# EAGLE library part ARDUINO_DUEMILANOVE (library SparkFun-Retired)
Arduino Duemilanove Shield Footprint Shield form compatible with the Arduino Duemilanove.
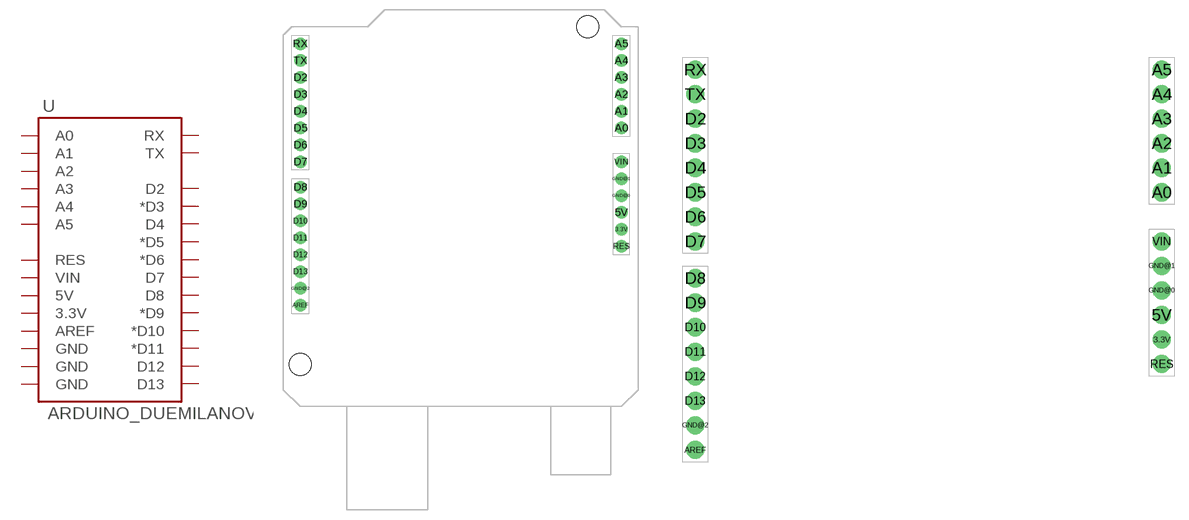
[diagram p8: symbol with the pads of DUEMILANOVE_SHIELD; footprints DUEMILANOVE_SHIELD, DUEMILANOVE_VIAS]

Designator prefix U

## ARDUINO_DUEMILANOVELABEL  [DUEMILANOVE_SHIELD]
3.3V  3.3V
5V  5V
A0  A0
A1  A1
A2  A2
A3  A3
A4  A4
A5  A5
AREF  AREF
D2  D2
D3  *D3
D4  D4
D5  *D5
D6  *D6
D7  D7
D8  D8
D9  *D9
D10  *D10
D11  *D11
D12  D12
D13  D13
GND@0  GND
GND@1  GND
GND@2  GND
RES  RES
RX  RX
TX  TX
VIN  VIN

## ARDUINO_DUEMILANOVENO_SILK  [DUEMILANOVE_VIAS]
Pads as for DUEMILANOVE_SHIELD

## ARDUINO_DUEMILANOVENOHOLES  [DUEMILANOVE_SHIELD_NOHOLES]
Pads as for DUEMILANOVE_SHIELD

## ARDUINO_DUEMILANOVELONGPADS  [DUEMILANOVE_SHIELD_LONGPADS]
Pads as for DUEMILANOVE_SHIELD

## ARDUINO_DUEMILANOVENOLABELS  [DUEMILANOVE_SHIELD_NOLABELS]
Pads as for DUEMILANOVE_SHIELD

## ARDUINO_DUEMILANOVENOHOLESORLABELS  [DUEMILANOVE_SHIELD_NOHOLES_NOLABELS]
Pads as for DUEMILANOVE_SHIELD

## Footprint DUEMILANOVE_SHIELD (pad centres in mm)
drill 1.016 pad 1.88: 3.3V 50.8,26.67; 5V 50.8,29.21; A0 50.8,41.91; A1 50.8,44.45; A2 50.8,46.99; A3 50.8,49.53; A4 50.8,52.07; A5 50.8,54.61; AREF 2.54,15.24; D2 2.54,49.53; D3 2.54,46.99; D4 2.54,44.45; D5 2.54,41.91; D6 2.54,39.37; D7 2.54,36.83; D8 2.54,33.02; D9 2.54,30.48; D10 2.54,27.94; D11 2.54,25.4; D12 2.54,22.86; D13 2.54,20.32; GND@0 50.8,31.75; GND@1 50.8,34.29; GND@2 2.54,17.78; RES 50.8,24.13; RX 2.54,54.61; TX 2.54,52.07; VIN 50.8,36.83
hole 3.302 at 45.72,57.15
hole 3.302 at 2.54,6.35

## Footprint DUEMILANOVE_VIAS (pad centres in mm)
drill 1.016 pad 1.88: 3.3V 50.8,13.97; 5V 50.8,16.51; A0 50.8,29.21; A1 50.8,31.75; A2 50.8,34.29; A3 50.8,36.83; A4 50.8,39.37; A5 50.8,41.91; AREF 2.54,2.54; D2 2.54,36.83; D3 2.54,34.29; D4 2.54,31.75; D5 2.54,29.21; D6 2.54,26.67; D7 2.54,24.13; D8 2.54,20.32; D9 2.54,17.78; D10 2.54,15.24; D11 2.54,12.7; D12 2.54,10.16; D13 2.54,7.62; GND@0 50.8,19.05; GND@1 50.8,21.59; GND@2 2.54,5.08; RES 50.8,11.43; RX 2.54,41.91; TX 2.54,39.37; VIN 50.8,24.13

## Footprint DUEMILANOVE_SHIELD_NOHOLES (pad centres in mm)
drill 1.016 pad 1.88: 3.3V 50.8,26.67; 5V 50.8,29.21; A0 50.8,41.91; A1 50.8,44.45; A2 50.8,46.99; A3 50.8,49.53; A4 50.8,52.07; A5 50.8,54.61; AREF 2.54,15.24; D2 2.54,49.53; D3 2.54,46.99; D4 2.54,44.45; D5 2.54,41.91; D6 2.54,39.37; D7 2.54,36.83; D8 2.54,33.02; D9 2.54,30.48; D10 2.54,27.94; D11 2.54,25.4; D12 2.54,22.86; D13 2.54,20.32; GND@0 50.8,31.75; GND@1 50.8,34.29; GND@2 2.54,17.78; RES 50.8,24.13; RX 2.54,54.61; TX 2.54,52.07; VIN 50.8,36.83

## Footprint DUEMILANOVE_SHIELD_LONGPADS (pad centres in mm)
drill 1.016 pad 1.88 long: 3.3V 50.8,26.67; 5V 50.8,29.21; A0 50.8,41.91; A1 50.8,44.45; A2 50.8,46.99; A3 50.8,49.53; A4 50.8,52.07; A5 50.8,54.61; AREF 2.54,15.24; D2 2.54,49.53; D3 2.54,46.99; D4 2.54,44.45; D5 2.54,41.91; D6 2.54,39.37; D7 2.54,36.83; D8 2.54,33.02; D9 2.54,30.48; D10 2.54,27.94; D11 2.54,25.4; D12 2.54,22.86; D13 2.54,20.32; GND@0 50.8,31.75; GND@1 50.8,34.29; GND@2 2.54,17.78; RES 50.8,24.13; RX 2.54,54.61; TX 2.54,52.07; VIN 50.8,36.83
hole 3.302 at 45.72,57.15
hole 3.302 at 2.54,6.35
